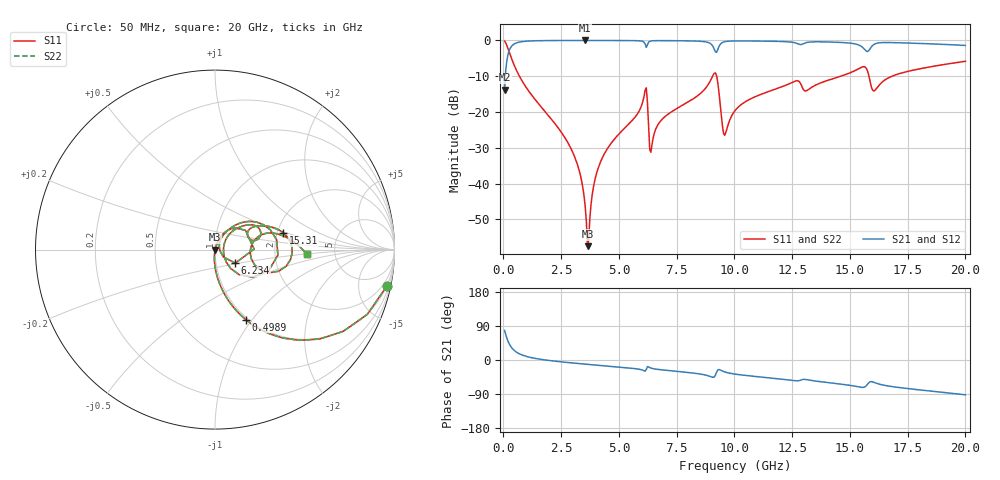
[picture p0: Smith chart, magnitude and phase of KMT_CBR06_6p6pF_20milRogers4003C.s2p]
! Data measured by Modelithics Inc. support@modelithics.com 813-866-6335
! KEMET CBR0603 6.6pF, Pad Width= 0.851mm, Pad Length= 0.64mm, Pad Gap= 0.62mm, 20mil Rogers 4003C substrate Data, January 2022
# hz S ma R 50
! 2 Port Network Data from SP1.SP block
! freq  magS11  angS11  magS21  angS21  magS12  angS12  magS22  angS22
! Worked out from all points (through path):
!   401 points, 50 MHz to 20 GHz, reference 50 ohm
!   highest |S21| = -0.01 dB at 3.541 GHz (marker M1); lowest = -13.8 dB at 50 MHz (marker M2)
!   group delay of S21, straight-line fit = 14.2 ps
!   lowest |S11| = -57.5 dB at 3.641 GHz (marker M3), VSWR 1.00, Z = 50.1 - j0.0942 ohm
!   |S11| at or under -10 dB: 692.3 MHz to 9.055 GHz (8.363 GHz wide, 172 % of centre); 9.231 GHz to 14.6 GHz (5.368 GHz wide, 45 % of centre); 15.82 GHz to 16.82 GHz (1 GHz wide, 6.13 % of centre)
!   |S22| runs from -57.5 to -0.2 dB; largest |S21 - S12| = 0
!   S11 on the Smith chart (normalised r, x): 50 MHz: 0.98, -9.43; 498.9 MHz: 0.98, -0.93; 6.234 GHz: 1.24, -0.19; 15.31 GHz: 2.16, +0.48; 20 GHz: 3.08, -0.20
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5e7  0.9787 -12.0  0.2049 78.0  0.2049 78.0  0.9787 -12.0
2.495e8  0.6898 -47.1  0.7235 42.8  0.7235 42.8  0.6898 -47.1
4.98875e8  0.4255 -66.3  0.9044 23.6  0.9044 23.6  0.4255 -66.3
2.74325e9  0.03958 -95.0  0.9981 -6.4  0.9981 -6.4  0.03958 -95.0
3.391625e9  0.01062 -94.3  0.9987 -10.1  0.9987 -10.1  0.01062 -94.3
3.54125e9  0.004735 -87.5  0.9988 -10.9  0.9988 -10.9  0.004735 -87.5
3.641e9  0.001337 -44.7  0.9988 -11.4  0.9988 -11.4  0.001337 -44.7
3.990125e9  0.01239 71.2  0.9986 -13.3  0.9986 -13.3  0.01239 71.2
4.33925e9  0.02499 72.0  0.9983 -15.1  0.9983 -15.1  0.02499 72.0
6.084875e9  0.1647 47.0  0.9452 -28.3  0.9452 -28.3  0.1647 47.0
6.2345e9  0.1361 -33.7  0.8684 -17.4  0.8684 -17.4  0.1361 -33.7
6.434e9  0.03567 47.1  0.9866 -22.1  0.9866 -22.1  0.03567 47.1
6.73325e9  0.06998 61.3  0.993 -25.1  0.993 -25.1  0.06998 61.3
9.12725e9  0.348 9.1  0.7544 -44.9  0.7544 -44.9  0.348 9.1
9.576125e9  0.04732 2.0  0.9598 -31.4  0.9598 -31.4  0.04732 2.0
1.0025e10  0.1044 46.5  0.9828 -37.2  0.9828 -37.2  0.1044 46.5
1.26185e10  0.269 27.7  0.9276 -54.6  0.9276 -54.6  0.269 27.7
1.336662e10  0.2236 30.6  0.9543 -54.3  0.9543 -54.3  0.2236 30.6
1.531175e10  0.3919 13.8  0.879 -70.2  0.879 -70.2  0.3919 13.8
1.605988e10  0.198 0.9  0.8864 -59.4  0.8864 -59.4  0.198 0.9
1.670825e10  0.3044 17.5  0.9339 -69.1  0.9339 -69.1  0.3044 17.5
2e10  0.5113 -2.7  0.8512 -91.8  0.8512 -91.8  0.5113 -2.7
